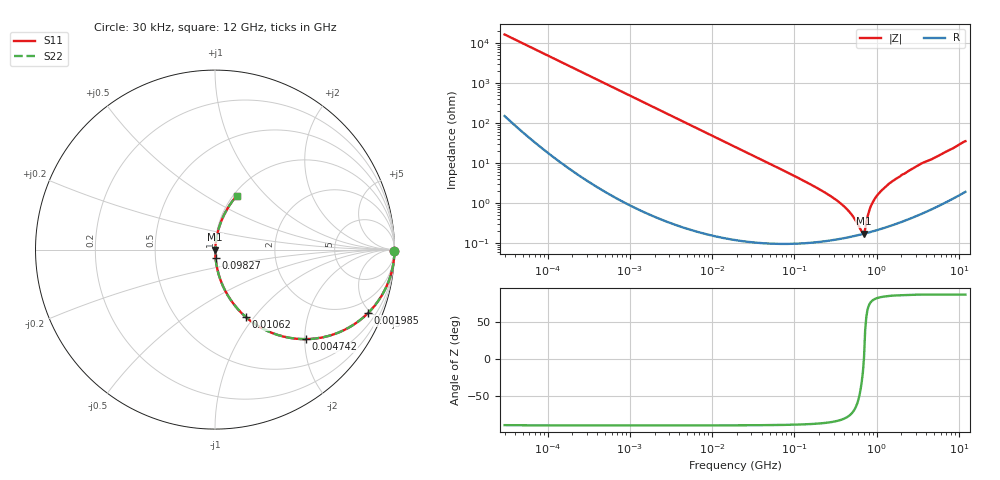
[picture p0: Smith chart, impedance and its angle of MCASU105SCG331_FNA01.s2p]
! MCASU105SCG331_FNA01  S-PARAMETER MODEL  ( General Type )
! Model Generated by TAIYO YUDEN Corporation (http://www.ty-top.com)
! Version 1.0
! TAIYO YUDEN Control No. 130207
! Copyright(c) 2013 TAIYO YUDEN CO.,LTD. All Rights Reserved.
! Product Description (link to TY-COMPAS)
! https://ds.yuden.co.jp/TYCOMPAS/or/detail?pn=MCASU105SCG331JFNA01&u=M
! Products Name : Multilayer Ceramic Capacitors
! Characteristics :
!  Capacitance : 330 pF , Rated Voltage : 50V , TCC : CG / C0G
!  Case Size : 1.0 x 0.5 / 0.039 x 0.02 [mm/inch] , Thickness : 0.5 / 0.02 [mm/inch]
!  (Conditions: Temperature = 25 degC , DC Bias Current/Voltage = 0A / 0V)
! External Node Assignments :
!  1  o---| |---o  2
! GND o---------o GND
! Frequency Range : 30000Hz  -  12GHz  [ 401 STEP ]
# MHz S RI R 50
! Freq[MHz].  S11 Real  S11 Imag  S21 Real  S21 Imag  S12 Real  S12 Imag  S22 Real  S22 Imag
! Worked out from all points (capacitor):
!   401 points, 30 kHz to 12 GHz, reference 50 ohm
!   read as one part in series: C = 331 pF near 32 kHz
!   lowest |Z| = 171 mohm at 702.6 MHz (marker M1)
!   series resonance near 700.6 MHz, so ESL is about 160 pH
!   S11 on the Smith chart (normalised r, x): 30 kHz: open; 1.985 MHz: 1.01, -4.85; 4.742 MHz: 1.00, -2.03; 10.62 MHz: 1.00, -0.91; 98.27 MHz: 1.00, -0.10; 12 GHz: 1.04, +0.69
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0.03  0.9999 -0.00624  9.63e-05 0.00624  9.63e-05 0.00624  0.9999 -0.00624
0.260295  0.997 -0.054  0.00305 0.054  0.00305 0.054  0.997 -0.054
0.75446  0.9757 -0.153  0.0243 0.153  0.0243 0.153  0.9757 -0.153
1.985138  0.8539 -0.3522  0.1461 0.3522  0.1461 0.3522  0.8539 -0.3522
2.258455  0.8188 -0.3842  0.1812 0.3842  0.1812 0.3842  0.8188 -0.3842
4.741653  0.507 -0.4988  0.493 0.4988  0.493 0.4988  0.507 -0.4988
10.61839  0.171 -0.3748  0.829 0.3748  0.829 0.3748  0.171 -0.3748
18.97367  0.0613 -0.2375  0.9387 0.2375  0.9387 0.2375  0.0613 -0.2375
39.83545  0.0152 -0.1184  0.9848 0.1184  0.9848 0.1184  0.0152 -0.1184
98.2684  0.00325 -0.0478  0.9967 0.0478  0.9967 0.0478  0.00325 -0.0478
164.6252  0.00178 -0.0276  0.9982 0.0276  0.9982 0.0276  0.00178 -0.0276
380.7415  0.00138 -0.00896  0.9986 0.00896  0.9986 0.00896  0.00138 -0.00896
508.9517  0.00148 -0.00457  0.9985 0.00457  0.9985 0.00457  0.00148 -0.00457
658.7456  0.00165 -0.000994  0.9983 0.000994  0.9983 0.000994  0.00165 -0.000994
702.6322  0.00171 5.39e-05  0.9983 -5.39e-05  0.9983 -5.39e-05  0.00171 5.39e-05
825.5698  0.00191 0.00682  0.9981 -0.00682  0.9981 -0.00682  0.00191 0.00682
909.4299  0.00208 0.0107  0.9979 -0.0107  0.9979 -0.0107  0.00208 0.0107
1068.55  0.00247 0.0173  0.9975 -0.0173  0.9975 -0.0173  0.00247 0.0173
1428.372  0.00355 0.0305  0.9965 -0.0305  0.9965 -0.0305  0.00355 0.0305
3303.507  0.013 0.0885  0.987 -0.0885  0.987 -0.0885  0.013 0.0885
6096.395  0.0345 0.1572  0.9655 -0.1572  0.9655 -0.1572  0.0345 0.1572
12000  0.1206 0.2996  0.8794 -0.2996  0.8794 -0.2996  0.1206 0.2996
